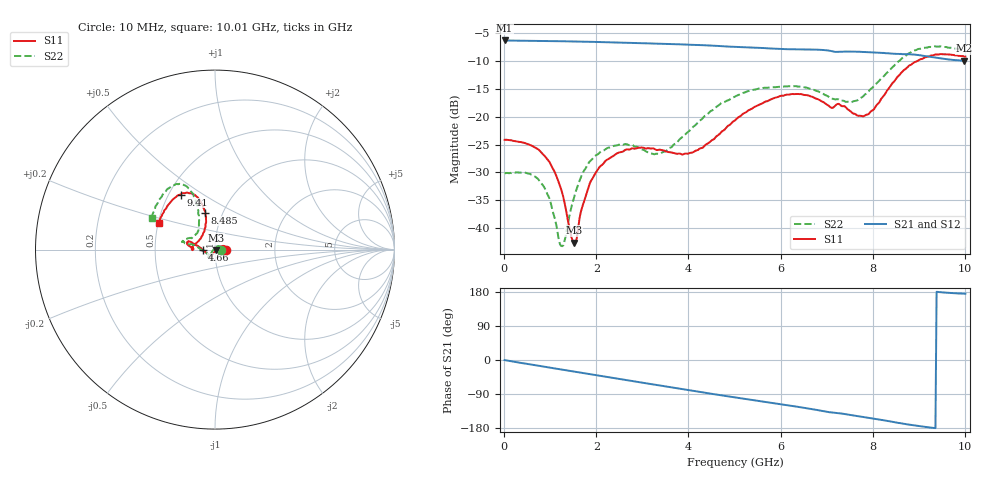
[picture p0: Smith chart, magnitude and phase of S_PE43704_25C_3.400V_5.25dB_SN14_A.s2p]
! Device ID: PE43704
! Dir: z:\PE43704\PE43704_Char_1_20130516\PE43704\AMB\3p400V\5p25dB
! Serial: 14
! Insertion: A
! Impedance: 50 ohm
! Temp: Amb
! VDD: 3.400V
! Attenuation Step: 5.25dB
! IDD: 1.139609e-01mA
#  Hz  S  RI  R  50
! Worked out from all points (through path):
!   401 points, 10 MHz to 10.01 GHz, reference 50 ohm
!   highest |S21| = -6.27 dB at 10 MHz (marker M1); lowest = -9.9 dB at 9.985 GHz (marker M2)
!   group delay of S21, straight-line fit = 52.8 ps
!   lowest |S11| = -42.6 dB at 1.51 GHz (marker M3), VSWR 1.01, Z = 50.5 - j0.503 ohm
!   |S11| at or under -10 dB: start of sweep to 8.96 GHz
!   |S22| runs from -43.3 to -7.3 dB; largest |S21 - S12| = 0.0034
!   S11 on the Smith chart (normalised r, x): 10 MHz: 1.13, +0.00; 4.66 GHz: 0.87, +0.00; 8.485 GHz: 0.83, +0.36; 9.41 GHz: 0.57, +0.40; 10.01 GHz: 0.50, +0.17
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1e7  0.0621 0.000231  0.4857 -0.00197  0.486 -0.00175  0.031 0.000317
7.85e8  0.0438 0.0215  0.4619 -0.1323  0.4619 -0.1321  0.0165 0.02
9.85e8  0.0345 0.0185  0.4507 -0.1636  0.4507 -0.1634  0.0086 0.0162
1.235e9  0.0206 0.00885  0.4331 -0.2021  0.4331 -0.2019  -0.00363 0.00587
1.31e9  0.0161 0.00532  0.4269 -0.213  0.4271 -0.2129  -0.00745 0.00169
1.51e9  0.00548 -0.00497  0.4097 -0.2414  0.4098 -0.2413  -0.0156 -0.00955
1.685e9  -0.00332 -0.0145  0.3931 -0.2653  0.3931 -0.2652  -0.0221 -0.0202
1.91e9  -0.0119 -0.0248  0.3692 -0.2936  0.3695 -0.2935  -0.0272 -0.0314
2.235e9  -0.0193 -0.0363  0.3316 -0.3307  0.3317 -0.3305  -0.0324 -0.041
3.36e9  -0.0255 -0.0437  0.1781 -0.4177  0.1786 -0.4175  -0.0377 -0.0271
4.035e9  -0.0401 -0.0251  0.0766 -0.4376  0.0771 -0.4377  -0.0757 -0.00216
4.66e9  -0.0692 6.39e-05  -0.0171 -0.4327  -0.0166 -0.4328  -0.1242 0.0272
5.01e9  -0.0914 0.017  -0.0644 -0.4209  -0.0642 -0.4212  -0.1492 0.0293
5.96e9  -0.1444 0.0463  -0.179 -0.3665  -0.1775 -0.3667  -0.1809 0.0431
6.685e9  -0.1495 0.0242  -0.2574 -0.3091  -0.2577 -0.3086  -0.1677 0.056
7.46e9  -0.1125 0.0297  -0.3122 -0.2273  -0.3121 -0.2274  -0.1049 0.0876
7.785e9  -0.0798 0.0614  -0.3327 -0.1896  -0.3328 -0.1905  -0.0897 0.1225
8.36e9  -0.0504 0.1756  -0.3522 -0.1165  -0.3516 -0.1181  -0.0986 0.2413
8.485e9  -0.054 0.2064  -0.3553 -0.0987  -0.3542 -0.1006  -0.108 0.2739
9.41e9  -0.192 0.3068  -0.3383 0.00228  -0.3378 0.00313  -0.2515 0.3455
9.985e9  -0.3079 0.1609  -0.3182 0.0279  -0.3194 0.0287  -0.3486 0.1849
1.001e10  -0.3129 0.1508  -0.3193 0.0282  -0.3211 0.0286  -0.3522 0.1765
